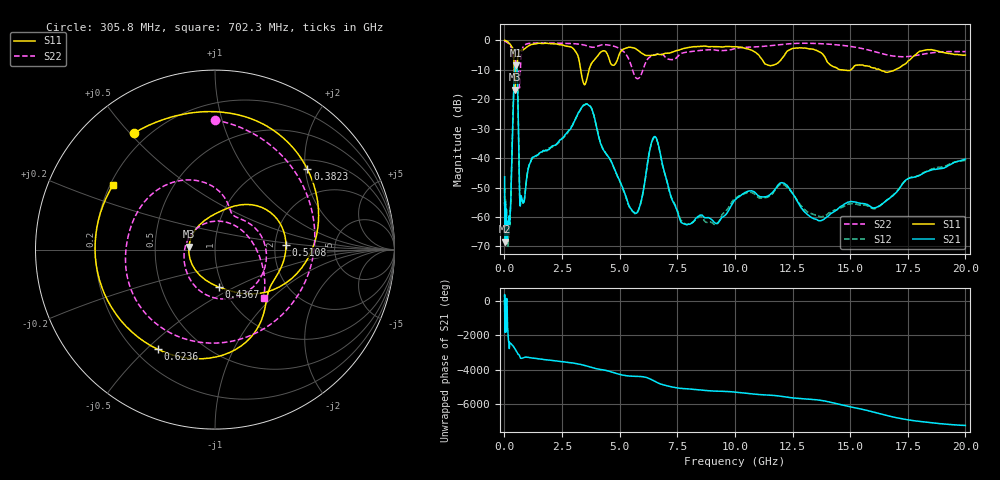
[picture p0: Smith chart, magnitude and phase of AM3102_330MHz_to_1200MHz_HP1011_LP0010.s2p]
! Date/Time: Tue, Sep 11, 2018 5:19 PM
! Network Analyzer: Agilent Technologies E8362B Rev: A.07.50.63
! Sweep from 0.010 to 20.000 GHz, 1601 Points, Sweep Type: LOG
! Power Supply: 4.949 V, 0.001 A
# Hz S DB R 50
!freq MagS11 AngS11 MagS21 AngS21 MagS12 AngS12 MagS22 AngS22
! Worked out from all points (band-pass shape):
!   1601 points, 10 MHz to 20 GHz, reference 50 ohm
!   highest |S21| = -8.53 dB at 484.8 MHz (marker M1); lowest = -68.4 dB at 42.59 MHz (marker M2)
!   |S21| within 3 dB of the highest: 429.8 MHz to 556.4 MHz (126.6 MHz wide, 25.7 % of centre)
!   lowest |S11| = -16.7 dB at 453.6 MHz (marker M3), VSWR 1.34, Z = 37.3 + j1.23 ohm
!   |S11| at or under -10 dB: 3.313 GHz to 3.67 GHz (357.9 MHz wide, 10.2 % of centre); 14.63 GHz to 15.03 GHz (402.5 MHz wide, 2.71 % of centre); 16.3 GHz to 16.95 GHz (647.3 MHz wide, 3.89 % of centre)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
!   |S22| runs from -16.1 to -0.2 dB; largest |S21 - S12| = 0.005
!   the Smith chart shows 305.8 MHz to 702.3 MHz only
!   S11 on the Smith chart (normalised r, x): 305.8 MHz: 0.15, +0.51; 382.3 MHz: 1.22, +2.05; 436.7 MHz: 0.95, -0.42; 510.8 MHz: 2.30, +0.15; 623.6 MHz: 0.29, -0.54; 702.3 MHz: 0.21, +0.28
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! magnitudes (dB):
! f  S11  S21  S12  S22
! 10 MHz  0.0  -46.3  -50.9  -0.2
! 35.55 MHz  0.0  -61.9  -63.1  -0.3
! 42.59 MHz  0.0  -68.4  -65.9  -0.3
! 126.4 MHz  -0.4  -63.9  -64.2  -0.7
! 223.5 MHz  -1.1  -62.7  -61.5  -1.3
! 305.8 MHz  -2.0  -45.6  -45.5  -2.8
! 382.3 MHz  -3.3  -22.0  -22.0  -5.7
! 436.7 MHz  -13.6  -10.6  -10.6  -5.9
! 447.2 MHz  -16.3  -9.6  -9.6  -6.1
! 453.6 MHz  -16.7  -9.2  -9.2  -6.2
! 484.8 MHz  -9.4  -8.5  -8.6  -6.7
! 510.8 MHz  -8.0  -8.6  -8.6  -8.5
! 623.6 MHz  -3.9  -35.2  -35.3  -11.9
! 702.3 MHz  -3.4  -54.5  -54.5  -8.3
! 1.59 GHz  -1.0  -37.9  -37.9  -0.9
! 3.634 GHz  -11.2  -21.9  -21.7  -2.0
! 5.652 GHz  -2.6  -58.6  -58.8  -12.1
! 6.518 GHz  -5.0  -32.6  -32.9  -4.9
! 7.92 GHz  -2.5  -62.6  -62.5  -4.0
! 12.03 GHz  -6.2  -48.3  -48.8  -1.4
! 13.81 GHz  -4.6  -61.0  -59.8  -1.2
! 20 GHz  -5.0  -40.3  -40.8  -3.8
